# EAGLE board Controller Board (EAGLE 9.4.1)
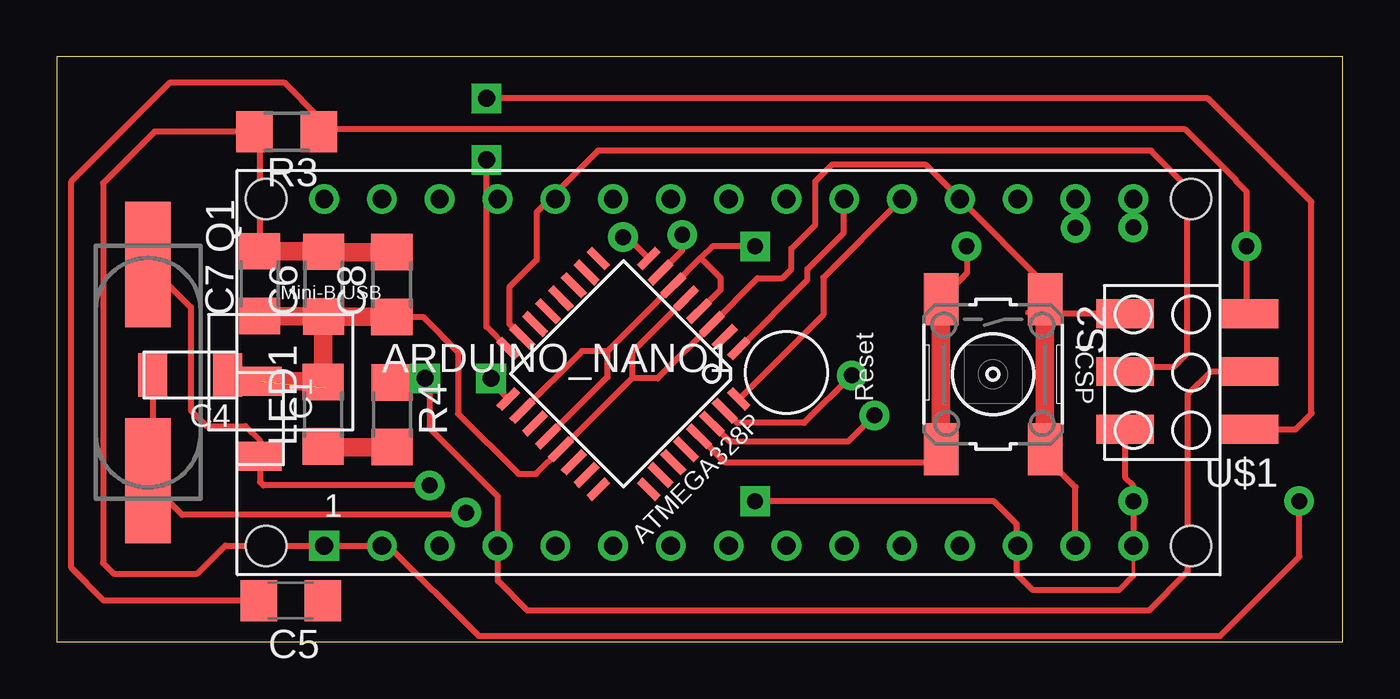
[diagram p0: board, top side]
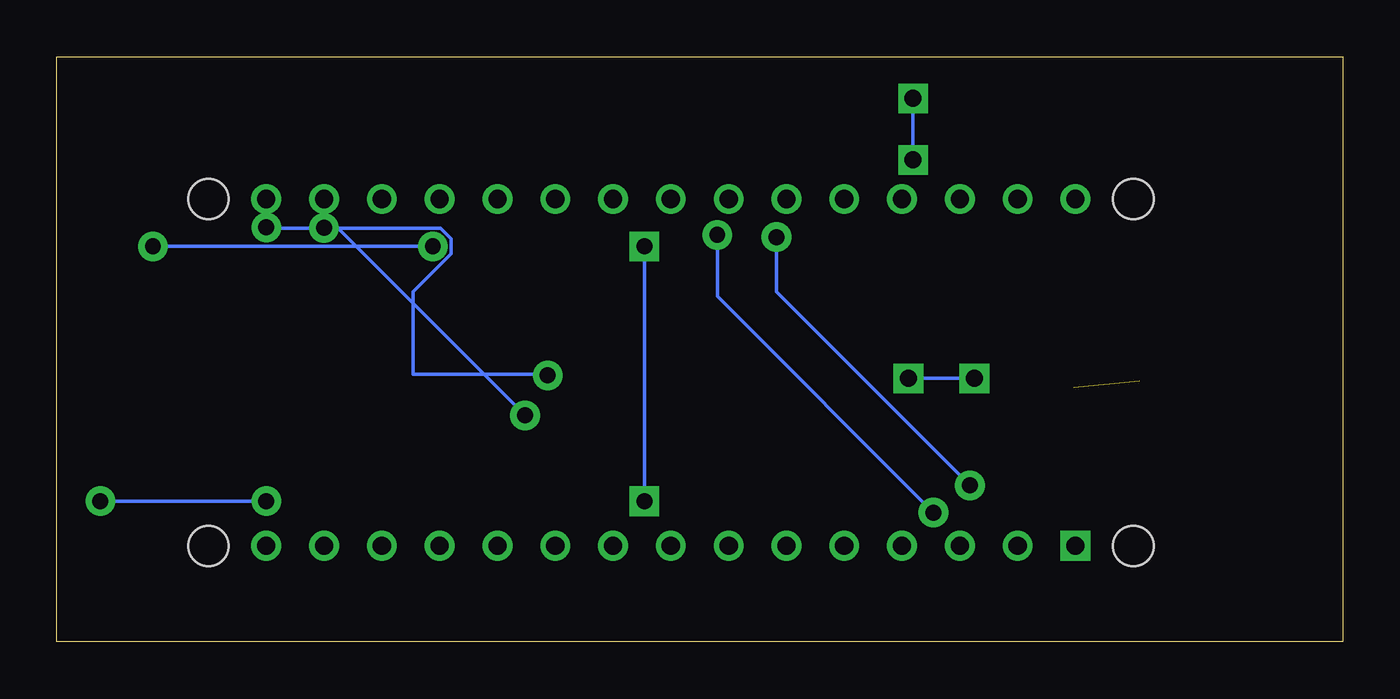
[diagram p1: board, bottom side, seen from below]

Size 56.5 x 25.7 mm. Coordinates in mm from the lower left corner, seen from the top.
Outline: 0,0 56.5,0 56.5,25.7 0,25.7 0,0
Copper layers (1*16): Top 0.035mm / dielectric 1.5mm / Bottom 0.035mm
Design rules "default": minimum track width 6mil, minimum drill 0.35mm, track to track 6mil, track to pad 6mil, pad to pad 6mil, via to via 6mil, smd to smd 6mil, copper to edge 40mil, drill to drill 6mil, minimum pad ring 10mil, minimum via ring 8mil, stop-mask expansion 4mil, vias tented up to drill 0mil, thermal gap 10mil

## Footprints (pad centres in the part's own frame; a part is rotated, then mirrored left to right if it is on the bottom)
ARDUINO_NANO = drill 0.8 square: 1 -20.32,-7.62 | drill 0.8: 2 -17.78,-7.62; 3 -15.24,-7.62; 4 -12.7,-7.62; 5 -10.16,-7.62; 6 -7.62,-7.62; 7 -5.08,-7.62; 8 -2.54,-7.62; 9 0,-7.62; 10 2.54,-7.62; 11 5.08,-7.62; 12 7.62,-7.62; 13 10.16,-7.62; 14 12.7,-7.62; 15 15.24,-7.62; 16 15.24,7.62; 17 12.7,7.62; 18 10.16,7.62; 19 7.62,7.62; 20 5.08,7.62; 21 2.54,7.62; 22 0,7.62; 23 -2.54,7.62; 24 -5.08,7.62; 25 -7.62,7.62; 26 -10.16,7.62; 27 -12.7,7.62; 28 -15.24,7.62; 29 -17.78,7.62; 30 -20.32,7.62 | hole 1.778: -22.86,-7.62; -22.86,7.62; 17.78,7.62; 17.78,-7.62
TQFP32-08THIN = smd 1.118 x 0.356: 1 -4.369,2.8; 8 -4.369,-2.8; 17 4.369,-2.8; 24 4.369,2.8 | smd 1.27 x 0.356: 2 -4.293,2; 3 -4.293,1.2; 4 -4.293,0.4; 5 -4.293,-0.4; 6 -4.293,-1.2; 7 -4.293,-2; 18 4.293,-2; 19 4.293,-1.2; 20 4.293,-0.4; 21 4.293,0.4; 22 4.293,1.2; 23 4.293,2 | smd 0.356 x 1.118: 9 -2.8,-4.369; 16 2.8,-4.369; 25 2.8,4.369; 32 -2.8,4.369 | smd 0.356 x 1.27: 10 -2,-4.293; 14 1.2,-4.293; 15 2,-4.293; 26 2,4.293; 27 1.2,4.293; 31 -2,4.293 | smd 0.35 x 1.27: 11 -1.2,-4.293; 12 -0.4,-4.293; 13 0.4,-4.293; 28 0.4,4.293; 29 -0.4,4.293; 30 -1.2,4.293
C1206FAB = smd 1.27 x 1.905: 1 -1.651,0; 2 1.651,0
C1206 = smd 1.6 x 1.8: 1 -1.4,0; 2 1.4,0
1206 = smd 1.6 x 1.803: 1 -1.422,0; 2 1.422,0
CSM-7X-DU = smd 5.5 x 2: 1 -4.75,0; 2 4.75,0
6MM_SWITCH = smd 2.286 x 1.524: 1 -3.302,2.286; 2 3.302,2.286; 3 -3.302,-2.286; 4 3.302,-2.286
2X03SMD = smd 2.54 x 1.27: 1 -2.54,2.54; 2 2.92,2.54; 3 -2.54,0; 4 2.92,0; 5 -2.54,-2.54; 6 2.92,-2.54

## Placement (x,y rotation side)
ARDUINO_NANO1  [ARDUINO_NANO]  32.06,11.84 0 top
ATMEGA328P  [TQFP32-08THIN]  24.9,11.78 225 top
C1  18/22pF  [C1206FAB]  8.93,9.81 270 top
C4  18/22 pF  [C1206FAB]  5.86,11.73 180 top
C5  .1uf  [C1206]  10.28,1.82 180 top
C6  1uf  [1206]  11.72,15.72 90 top
C7  .1uf  [1206]  8.92,15.74 90 top
C8  10uf  [1206]  14.72,15.7 90 top
LED1  [1206]  11.7,10 90 top
Q1  16Mhz  [CSM-7X-DU]  4.01,11.83 270 top
R3  10k  [1206]  10.1,22.42 180 top
R4  499  [1206]  14.74,9.98 270 top
S2  [6MM_SWITCH]  41.14,11.76 270 top
U$1  AVRISPSMD  [2X03SMD]  49.86,11.88 180 top

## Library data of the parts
ARDUINO_NANO1 = ArduinoNanoV30
ATMEGA328P C1 C4 = 1_fab
C5 = rcl
C6-C8 LED1 R3 R4 S2 = ng
Q1 = crystal; OC_FARNELL: unknown; OC_NEWARK: unknown
U$1 = fab

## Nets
5V: ARDUINO_NANO1.12
GND: ARDUINO_NANO1.14 ARDUINO_NANO1.19 ATMEGA328P.3 ATMEGA328P.5 ATMEGA328P.21 C1.1 C4.1 C6.1 C7.1 C8.1 LED1.2 S2.1 S2.2 U$1.6
N$1: ATMEGA328P.8 C1.2 Q1.1
N$2: ATMEGA328P.7 C4.2 Q1.2
N$16: ATMEGA328P.15 U$1.4
N$19: ATMEGA328P.16 U$1.1
N$20: ATMEGA328P.17 R4.1 U$1.3
N$21: LED1.1 R4.2
N$25: C5.1
N$26: ARDUINO_NANO1.17 ATMEGA328P.30
N$27: ARDUINO_NANO1.21 ATMEGA328P.1
N$28: ARDUINO_NANO1.20 ATMEGA328P.32
N$29: ARDUINO_NANO1.16 ATMEGA328P.31
RST1: ATMEGA328P.29 C5.2 R3.1 S2.3 S2.4 U$1.5
VCC: ARDUINO_NANO1.15 ATMEGA328P.4 ATMEGA328P.6 ATMEGA328P.18 ATMEGA328P.20 C6.2 C7.2 C8.2 R3.2 U$1.2

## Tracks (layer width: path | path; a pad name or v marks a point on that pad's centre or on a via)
GND  (1 unrouted)
  Top 0.152: 11.78,14.32 11.68,14.32 11.7,14.3 | 11.78,14.32 11.76,14.34 C6.1 | 11.78,14.32 11.82,14.28 11.88,14.28 11.9,14.26 | 14.73,14.27 C8.1 | 43.24,14.42 43.18,14.48 43.01,14.65 S2.1 | 42.68,14.48 42.63,14.43 | 11.82,11.16 11.9,11.08 | 25.28,11.58 25.27,11.58 | C4.1 8.66,11.73 C1.1
  Top 0.254: U$1.6 43.24,14.42 | S2.2 43.43,8.13 44.76,6.8 ARDUINO_NANO1.14 | 42.68,14.48 43.18,14.48 | S2.1 43.43,15.71 ARDUINO_NANO1.19 38.16,20.98 34.08,20.98 33.33,20.23 33.33,18.33 32.28,17.28 32.28,16.38 31.88,15.98 30.8,15.98 ATMEGA328P.3 26.4,11.58 25.28,11.58 25.28,12.73 ATMEGA328P.5 | 25.27,11.58 ATMEGA328P.21 21.07,7.38 20.28,7.38 17.63,10.03 17.63,12.73 16.08,14.28 C8.1
  Top 0.813: C7.1 11.68,14.32 | C8.1 11.88,14.28 | C1.1 11.66,11.46 LED1.2 11.7,14.3 | S2.1 S2.2
N$1  (via drill 0.7 pad 1.3)
  Top 0.152: 25.08,17.78 v24.88,17.78
  Top 0.254: Q1.1 5.88,14.71 5.88,10.18 6.58,9.48 8.28,9.48 8.93,8.83 C1.2 8.93,7.03 9.08,6.88 v16.38,6.88 | ATMEGA328P.8 25.08,17.78
  Bottom 0.152: v16.38,6.88 24.88,15.38 v24.88,17.78
N$2  (via drill 0.7 pad 1.3)
  Top 0.152: 4.21,7.28 Q1.2
  Top 0.254: Q1.2 5.51,5.58 17.88,5.58 v17.98,5.68 | v27.48,17.88 27.48,17.19 ATMEGA328P.7 | C4.2 4.21,7.28
  Bottom 0.152: v17.98,5.68 27.48,15.18 v27.48,17.88
N$16
  Top 0.152: U$1.4 47.14,12.08
  Top 0.254: ATMEGA328P.15 19.88,13.97 19.88,15.58 21.08,16.78 21.08,18.88 23.78,21.58 48.08,21.58 49.68,19.98 49.68,12.68 49.08,12.08 47.14,12.08
N$19  (via drill 0.75 pad 1.3)
  Top 0.152: 55.13,10.03 55.18,10.08
  Top 0.254: ATMEGA328P.16 18.88,13.84 v18.88,21.18 | U$1.1 54.44,9.34 55.13,10.03 55.13,19.33 50.58,23.88 v18.88,23.88
  Bottom 0.152: v18.88,23.88 v18.88,21.18
N$20  (via drill 0.75 pad 1.3)
  Top 0.152: 19.08,11.42 v19.08,11.58
  Top 0.254: R4.1 16,11.4 v16.18,11.58 16.18,11.28 16.38,11.08 16.38,9.38 19.38,6.38 19.38,2.68 20.68,1.38 47.98,1.38 49.68,3.08 49.68,10.88 50.68,11.88 U$1.3 | ATMEGA328P.17 19.08,11.42
  Bottom 0.152: v19.08,11.58 v16.18,11.58
N$21
  Top 0.152: R4.2 14.76,8.58
  Top 0.813: LED1.1 11.72,8.56 R4.2
N$26  (via drill 0.7 pad 1.3)
  Top 0.254: ARDUINO_NANO1.17 v44.76,18.19 | v35.92,9.96 34.77,8.8 29.58,8.8 ATMEGA328P.30
  Bottom 0.152: v44.76,18.19 44.17,18.19 v35.93,9.95 v35.92,9.96
N$27
  Top 0.254: ARDUINO_NANO1.21 34.58,19.44 34.58,17.98 32.98,16.38 32.98,15.9 ATMEGA328P.1
N$28
  Top 0.254: ATMEGA328P.32 33.68,14.38 33.68,16 ARDUINO_NANO1.20
N$29  (via drill 0.7 pad 1.3)
  Top 0.254: v34.93,11.71 32.84,9.62 29.89,9.62 ATMEGA328P.31 | ARDUINO_NANO1.16 v47.3,18.21
  Bottom 0.152: v47.3,18.21 47.27,18.18 39.65,18.18 39.18,17.71 39.18,17.05 40.85,15.37 40.85,11.76 34.98,11.76 v34.93,11.71
RST1  (via drill 0.7 pad 1.3)
  Top 0.152: U$1.5 52.28,14.54 | 51.82,20.28 51.82,20.24 | 11.62,22.52 R3.1 11.52,23.04 | S2.4 38.28,7.88 | S2.3 38.85,15.35
  Top 0.254: 52.28,14.54 v52.28,17.38 52.28,19.78 51.82,20.24 | 11.62,22.52 49.58,22.52 51.82,20.28 | C5.2 2.06,1.82 0.63,3.25 0.63,20.23 4.98,24.58 9.98,24.58 11.52,23.04 | ATMEGA328P.29 29.37,7.88 38.28,7.88 | v39.98,17.38 39.98,16.19 S2.3
  Top 0.813: S2.3 S2.4
  Bottom 0.152: v39.98,17.38 v52.28,17.38
VCC  (via drill 0.7 pad 1.3)
  Top 0.152: 11.7,17.16 C6.2 11.74,17.12 | 30.78,6.08 v30.68,6.18 | ARDUINO_NANO1.15 47.3,2.9 | R3.2 8.92,22.18 | 54.6,6.14 54.59,6.15 v54.59,6.19
  Top 0.254: U$1.2 46.94,7.22 47.3,6.86 v47.3,6.19 ARDUINO_NANO1.15 | ATMEGA328P.4 29.18,15.49 29.18,15.98 28.29,16.87 | 24.2,12.78 ATMEGA328P.6 28.29,16.87 | ATMEGA328P.18 23.07,12.78 24.2,12.78 | ATMEGA328P.20 24.2,11.65 24.2,12.78 | 28.29,16.87 28.8,17.38 v30.68,17.38 | 47.3,2.9 46.68,2.28 42.88,2.28 42.18,2.98 42.18,5.18 41.18,6.18 v30.68,6.18 | 8.92,22.18 C7.2 | R3.2 4.29,22.42 2.03,20.16 2.03,3.46 2.49,3 6.17,3 7.4,4.23 14.56,4.23 18.52,0.27 51.12,0.27 54.6,3.75 54.6,6.14
  Top 0.813: C7.2 11.7,17.16 | C8.2 11.74,17.12
  Bottom 0.152: v30.68,17.38 v30.68,6.18 | v54.59,6.19 v47.3,6.19 v47.29,6.19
